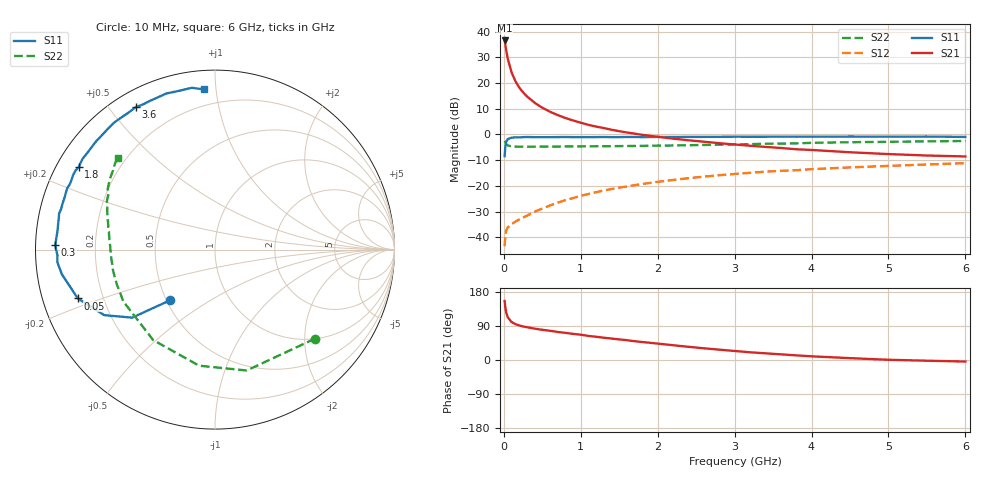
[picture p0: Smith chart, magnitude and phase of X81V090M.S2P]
! SIEMENS Small Signal Semiconductors
! BFP136W
! Si NPN RF Bipolar Junction Transistor in SOT343
! VCE = 1 V  IC = 90 mA
! Common Emitter S-Parameters:  September  1994
# GHz  S  MA  R  50
!  f  S11  S21  S12  S22
! GHz  MAG  ANG  MAG  ANG  MAG  ANG  MAG  ANG
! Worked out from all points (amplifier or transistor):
!   40 points, 10 MHz to 6 GHz, reference 50 ohm
!   highest |S21| = 36.6 dB at 10 MHz (marker M1)
!   |S21| within 3 dB of that: start of sweep to 26.51 MHz
!   unconditionally stable (mu >= 1): 428.2 MHz to 3.451 GHz; 3.708 GHz to 3.969 GHz; 5.748 GHz to end of sweep
!   at 200 MHz: K = 0.73, MSG = 25.7 dB, |S12| = -33.1 dB
!   at 1.5 GHz: K = 1.14, MAG = 8.7 dB, |S12| = -20.7 dB
!   at 6 GHz: K = 1.03, MAG = 0.3 dB, |S12| = -11.2 dB
!   S11 on the Smith chart (normalised r, x): 10 MHz: 0.52, -0.34; 50 MHz: 0.11, -0.17; 300 MHz: 0.06, +0.01; 1.8 GHz: 0.06, +0.28; 3.6 GHz: 0.06, +0.59; 6 GHz: 0.10, +0.93
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0.01  0.3767 -131.5  67.44 155.9  0.0067 63.4  0.746 -41.7
0.02  0.5973 -140.6  54.93 137.7  0.0108 50.6  0.6963 -75.3
0.03  0.7174 -149.4  44.29 125.9  0.0134 42.4  0.6528 -97.8
0.05  0.8113 -160.4  30.23 113.0  0.0155 33.7  0.6103 -124.4
0.1  0.8647 -170.9  16.2 100.4  0.018 33.6  0.5868 -150.4
0.15  0.8808 -175.4  10.93 94.7  0.0201 37.5  0.5801 -160.4
0.2  0.8782 -177.9  8.182 91.2  0.0222 41.0  0.5793 -165.6
0.25  0.8858 179.8  6.596 88.5  0.0242 44.4  0.5797 -169.0
0.3  0.8906 178.4  5.51 86.6  0.0262 48.1  0.5782 -171.3
0.4  0.8851 175.0  4.145 82.8  0.0314 52.5  0.5796 -174.4
0.5  0.8836 172.9  3.307 79.7  0.0362 55.7  0.5803 -176.6
0.6  0.8853 171.0  2.765 77.1  0.0415 57.8  0.5812 -178.2
0.8  0.8915 167.0  2.091 71.6  0.0526 60.7  0.5832 179.4
1.1  0.887 160.9  1.536 63.5  0.0694 61.5  0.5875 176.6
1.4  0.8875 156.0  1.235 56.6  0.0867 60.5  0.5915 174.0
1.8  0.8871 148.8  0.984 47.4  0.1086 57.9  0.5987 170.5
2.2  0.8923 142.1  0.829 39.0  0.1301 54.5  0.6098 167.2
3.2  0.9024 125.2  0.603 20.4  0.1791 44.4  0.6474 157.9
3.6  0.9083 119.0  0.546 15.0  0.1956 40.3  0.6645 154.3
4.5  0.9109 107.3  0.45 4.9  0.2285 31.6  0.706 146.1
5.5  0.9108 98.2  0.389 -1.9  0.2604 23.5  0.7346 139.4
6  0.8946 93.9  0.373 -4.1  0.2764 19.2  0.7453 136.6
